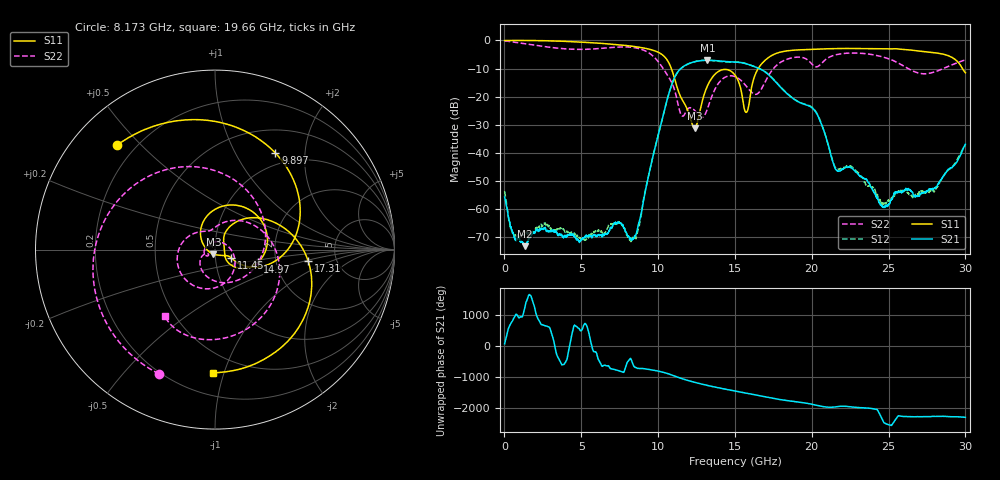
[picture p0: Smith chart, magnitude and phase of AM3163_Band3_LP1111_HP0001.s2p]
!Agilent Technologies,E8364B,MY43040894,A.07.50.67
!Agilent E8364B: A.07.50.67
!Date: Thursday, August 20, 2020 12:15:07
!Correction: S11(Full 2 Port(1,2))
!S21(Full 2 Port(1,2))
!S12(Full 2 Port(1,2))
!S22(Full 2 Port(1,2))
!S2P File: Measurements: S11, S21, S12, S22:
# Hz S  dB  R 50
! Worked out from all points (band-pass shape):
!   3201 points, 10 MHz to 30 GHz, reference 50 ohm
!   highest |S21| = -7.06 dB at 13.21 GHz (marker M1); lowest = -73.3 dB at 1.322 GHz (marker M2)
!   |S21| within 3 dB of the highest: 11.47 GHz to 16.6 GHz (5.128 GHz wide, 36.5 % of centre)
!   lowest |S11| = -31.3 dB at 12.37 GHz (marker M3), VSWR 1.06, Z = 49 - j2.54 ohm
!   |S11| at or under -10 dB: 10.86 GHz to 16.52 GHz (5.655 GHz wide, 41.3 % of centre); 29.81 GHz to end of sweep
!   |S22| runs from -27.4 to -0.1 dB; largest |S21 - S12| = 0.013
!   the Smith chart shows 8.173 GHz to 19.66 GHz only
!   S11 on the Smith chart (normalised r, x): 8.173 GHz: 0.13, +0.43; 9.897 GHz: 0.82, +1.47; 11.45 GHz: 1.19, -0.11; 14.97 GHz: 1.60, -0.24; 17.31 GHz: 3.09, -0.53; 19.66 GHz: 0.35, -0.92
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1e7  -0.02 -1.8  -55.79 82.5  -53.71 30.4  -0.14 -5.0
1.322062e9  -0.01 -36.2  -73.33 165.6  -68.97 -116.0  -1.18 -87.3
2.952769e9  -0.14 -80.6  -68.01 -129.5  -66.67 -46.5  -2.43 -179.0
5.014581e9  -0.60 -135.3  -71.00 159.6  -70.54 -171.9  -3.20 71.7
6.570312e9  -1.14 -177.7  -68.95 104.5  -68.53 -26.7  -2.69 -16.1
8.172903e9  -1.97 133.0  -70.55 -42.1  -71.19 168.1  -2.39 -114.2
9.044488e9  -2.67 100.0  -57.30 2.5  -56.83 5.1  -3.43 -178.1
9.897328e9  -3.95 58.0  -36.02 -65.9  -36.08 -65.3  -6.83 96.1
1.000979e10  -4.22 51.2  -33.52 -77.5  -33.60 -77.3  -7.57 81.1
1.145306e10  -19.92 -27.3  -10.14 56.4  -10.17 56.9  -25.94 -154.5
1.23715e10  -31.25 -109.1  -7.58 -78.2  -7.58 -77.9  -24.89 176.4
1.321497e10  -16.16 118.1  -7.06 179.8  -7.06 179.3  -24.28 33.5
1.496751e10  -12.08 -16.5  -7.68 3.7  -7.75 5.4  -12.81 -150.7
1.5005e10  -12.34 -19.1  -7.69 0.1  -7.75 1.8  -12.88 -153.8
1.575475e10  -25.60 10.4  -8.35 -72.8  -8.29 -72.0  -16.38 145.0
1.731048e10  -5.64 -6.9  -12.83 136.8  -12.71 137.7  -11.46 27.6
1.966282e10  -3.26 -91.1  -23.03 -34.0  -22.89 -33.1  -6.68 -127.3
2.000958e10  -3.20 -100.0  -23.94 -67.0  -23.77 -66.5  -8.42 -137.6
2.157468e10  -2.90 -136.7  -46.03 -150.7  -45.60 -148.1  -5.11 -159.5
2.500479e10  -3.00 144.6  -58.31 -11.9  -56.88 -167.0  -6.54 67.7
2.740399e10  -4.01 78.1  -53.82 -104.2  -54.19 130.3  -11.89 -88.0
3e10  -11.52 -27.7  -37.01 -128.6  -37.58 -128.9  -6.97 130.2
